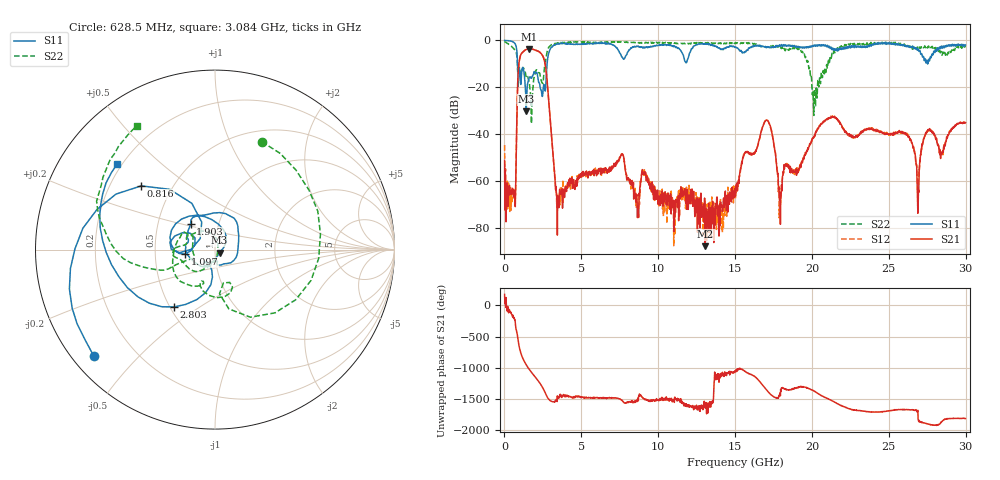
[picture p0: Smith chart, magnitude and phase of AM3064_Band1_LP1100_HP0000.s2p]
# Hz S DB R 50.0
!freq dBS11 angS11 dBS21 angS21 dBS12 angS12 dBS22 angS22
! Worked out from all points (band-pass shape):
!   1600 points, 10 MHz to 29.98 GHz, reference 50 ohm
!   highest |S21| = -3.63 dB at 1.622 GHz (marker M1); lowest = -87.6 dB at 13.06 GHz (marker M2)
!   |S21| within 3 dB of the highest: 1.036 GHz to 2.494 GHz (1.458 GHz wide, 82.6 % of centre)
!   lowest |S11| = -30.1 dB at 1.416 GHz (marker M3), VSWR 1.06, Z = 52.6 - j1.89 ohm
!   |S11| at or under -10 dB: 848.8 MHz to 2.773 GHz (1.924 GHz wide, 106 % of centre); 27.52518 GHz to 27.52957 GHz (4.392 MHz wide, 0.016 % of centre)
!   |S22| runs from -35.5 to -0.4 dB; largest |S21 - S12| = 0.01
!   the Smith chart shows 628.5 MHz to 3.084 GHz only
!   S11 on the Smith chart (normalised r, x): 628.5 MHz: 0.06, -0.38; 816 MHz: 0.33, +0.34; 1.097 GHz: 0.71, -0.04; 1.903 GHz: 0.73, +0.22; 2.803 GHz: 0.53, -0.40; 3.084 GHz: 0.18, +0.36
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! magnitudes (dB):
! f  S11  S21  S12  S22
! 10 MHz  0.0  -51.1  -44.6  -0.4
! 628.5 MHz  -0.9  -66.4  -63.7  -3.7
! 816 MHz  -5.3  -30.6  -30.5  -7.4
! 1.097 GHz  -15.4  -5.7  -5.7  -14.1
! 1.416 GHz  -30.1  -3.9  -3.8  -15.8
! 1.622 GHz  -15.8  -3.6  -3.6  -18.3
! 1.903 GHz  -14.1  -3.9  -3.9  -16.4
! 2.803 GHz  -8.1  -19.4  -19.4  -4.3
! 3.084 GHz  -2.8  -43.1  -42.4  -1.8
! 3.515 GHz  -1.5  -67.5  -67.0  -1.1
! 5.015 GHz  -1.4  -56.6  -56.7  -0.7
! 7.62 GHz  -6.9  -48.6  -48.3  -0.7
! 10 GHz  -2.1  -69.8  -65.7  -1.0
! 13.06 GHz  -1.6  -87.6  -80.7  -1.1
! 15 GHz  -2.8  -64.1  -62.5  -1.4
! 17.01 GHz  -3.0  -34.0  -34.0  -2.9
! 17.93 GHz  -2.1  -64.7  -68.9  -2.7
! 19.99 GHz  -2.8  -42.8  -42.8  -18.3
! 25 GHz  -1.0  -40.0  -39.8  -1.1
! 26.89 GHz  -3.8  -73.6  -67.0  -3.4
! 27.53 GHz  -10.0  -38.5  -38.4  -3.1
! 29.98 GHz  -1.9  -35.0  -34.9  -3.0
